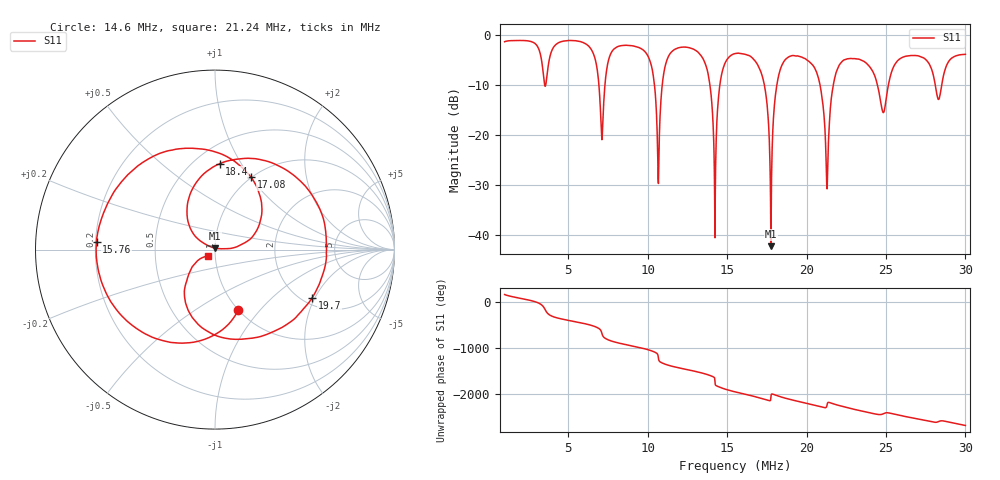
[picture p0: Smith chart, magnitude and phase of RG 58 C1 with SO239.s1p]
! Format: Frequency Z-real Z-imaginary (normalized to 50 Ohm)
# MHz Z RI R 50
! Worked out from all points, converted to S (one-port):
!   1451 points, 1 MHz to 30 MHz, reference 50 ohm
!   lowest |S11| = -42.2 dB at 17.76 MHz (marker M1), VSWR 1.02, Z = 50.2 + j0.76 ohm
!   |S11| at or under -10 dB: 17.35 MHz to 18.13 MHz (780 kHz wide, 4.4 % of centre); 20.85 MHz to 21.68 MHz (830.3 kHz wide, 3.9 % of centre); 24.47 MHz to 25.15 MHz (682.7 kHz wide, 2.75 % of centre)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
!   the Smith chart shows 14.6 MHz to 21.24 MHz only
!   S11 on the Smith chart (normalised r, x): 14.6 MHz: 0.99, -0.78; 15.76 MHz: 0.20, +0.03; 17.08 MHz: 0.99, +1.01; 18.4 MHz: 0.65, +0.81; 19.7 MHz: 2.26, -1.91; 21.24 MHz: 0.92, -0.06
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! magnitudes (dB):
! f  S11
! 1 MHz  -1.3
! 3.56 MHz  -10.2
! 4.64 MHz  -1.2
! 6.5 MHz  -3.1
! 7.12 MHz  -20.9
! 8.26 MHz  -2.1
! 10.06 MHz  -4.4
! 10.68 MHz  -29.7
! 11.1 MHz  -6.2
! 11.88 MHz  -2.6
! 13.62 MHz  -5.6
! 14.22 MHz  -32.8
! 14.6 MHz  -8.8
! 15.5 MHz  -3.7
! 15.76 MHz  -3.6
! 17.08 MHz  -6.9
! 17.76 MHz  -42.2
! 18.4 MHz  -6.4
! 19.14 MHz  -4.0
! 19.7 MHz  -4.4
! 20.74 MHz  -8.4
! 21.24 MHz  -25.8
! 21.82 MHz  -8.0
! 22.76 MHz  -4.6
! 24.84 MHz  -15.5
! 26.38 MHz  -4.1
! 28.3 MHz  -12.8
! 30 MHz  -3.8
